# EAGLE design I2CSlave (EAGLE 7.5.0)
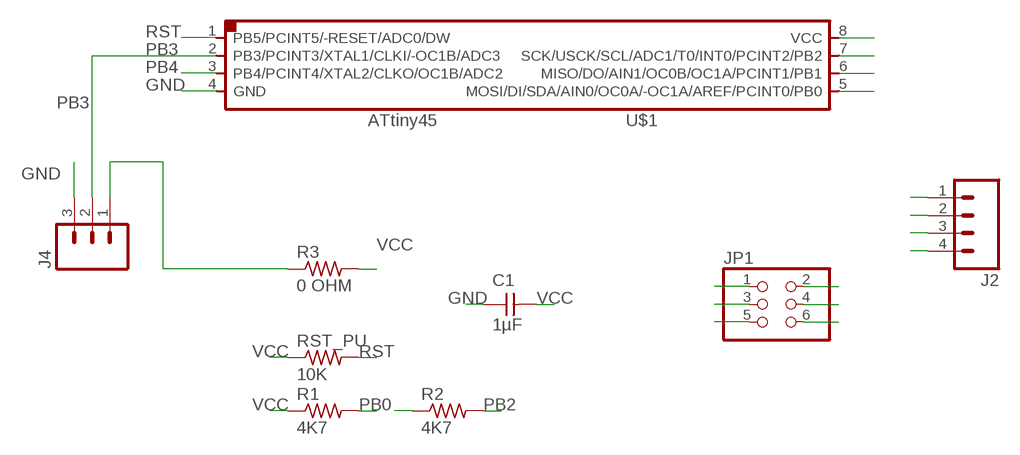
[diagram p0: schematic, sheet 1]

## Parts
C1  1µF  CAP-UNPOLARIZEDFAB  [C1206FAB]
J2  M04LONGPADS  [1X04_LONGPADS]
J4  M03LONGPADS  [1X03_LONGPADS]
JP1  PINHD-2X3-SMD  [2X03SMD]
R1  4K7  RES-US1206FAB  [R1206FAB]
R2  4K7  RES-US1206FAB  [R1206FAB]
R3  0 OHM  RES-US1206FAB  [R1206FAB]
RST_PU  10K  RES-US1206FAB  [R1206FAB]
U$1  ATTINY45SI  [SOIC8]

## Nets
GND: C1.1 J2.4 J4.3 JP1.6 U$1.4(GND)
MISO: JP1.1 U$1.6(MISO/DO/AIN1/OC0B/OC1A/PCINT1/PB1)
N$1: J4.1 R3.1
PB0: J2.2 JP1.4 R1.2 U$1.5(MOSI/DI/SDA/AIN0/OC0A/-OC1A/AREF/PCINT0/PB0)
PB2: J2.3 JP1.3 R2.2 U$1.7(SCK/USCK/SCL/ADC1/T0/INT0/PCINT2/PB2)
PB3: J4.2 U$1.2(PB3/PCINT3/XTAL1/CLKI/-OC1B/ADC3)
PB4: U$1.3(PB4/PCINT4/XTAL2/CLKO/OC1B/ADC2)
RST: JP1.5 RST_PU.2 U$1.1(PB5/PCINT5/-RESET/ADC0/DW)
VCC: C1.2 J2.1 JP1.2 R1.1 R2.1 R3.2 RST_PU.1 U$1.8(VCC)

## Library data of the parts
C1 = fab:CAP-UNPOLARIZED
J2 = SparkFun-Connectors:M04: Header 4 Standard 4-pin 0.1" header. Use with straight break away headers (SKU : PRT-00116), right angle break away headers (PRT-00553), swiss pins (PRT-00743), machine pins (PRT-00117), and female headers (PRT-00115). Molex polarized connector foot print use with SKU : PRT-08231 with associated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; PROD_ID: CONN-09696
J4 = SparkFun-Connectors:M03: Header 3 Standard 3-pin 0.1" header. Use with straight break away headers (SKU : PRT-00116), right angle break away headers (PRT-00553), swiss pins (PRT-00743), machine pins (PRT-00117), and female headers (PRT-00115). Molex polarized connector foot print use with SKU : PRT-08232 with associated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
JP1 = fab:PINHD-2X3-SMD: PIN HEADER
R1-R3 RST_PU = fab:RES-US: Resistor (US Symbol)
U$1 = fab:ATTINY45

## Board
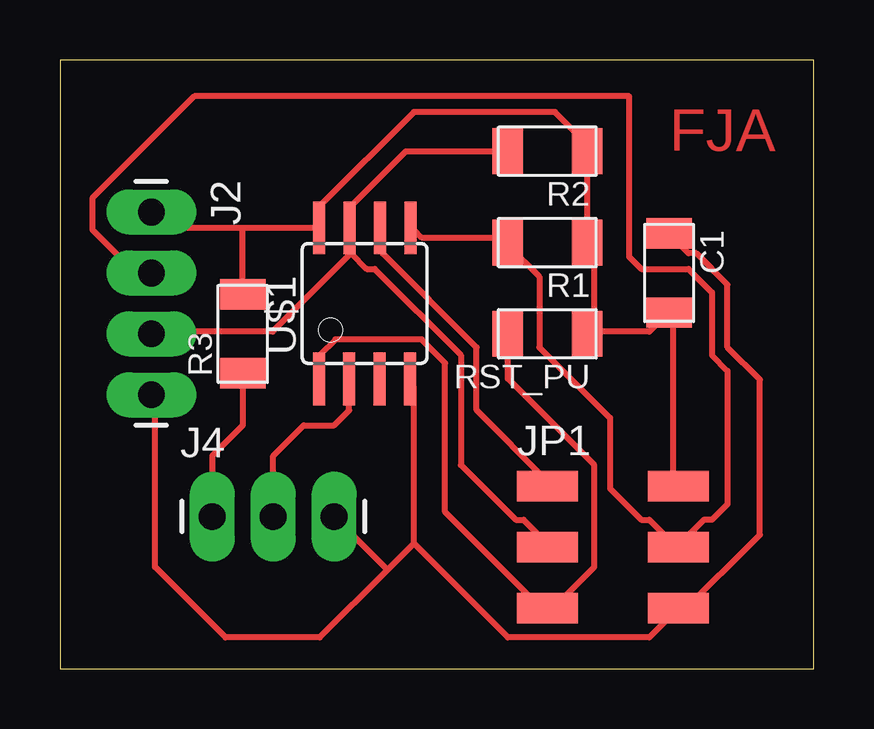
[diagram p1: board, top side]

Size 31.42 x 25.39 mm. Coordinates in mm from the lower left corner, seen from the top.
Outline: 0,0 31.42,0 31.42,25.39 0,25.39 0,0
Copper layers (1*16): Top 0.035mm / dielectric 1.5mm / Bottom 0.035mm
Design rules "default *": minimum track width 10mil, minimum drill 24mil, track to track 0.4mm, track to pad 0.4mm, pad to pad 0.4mm, via to via 0.4mm, smd to smd 8mil, copper to edge 40mil, drill to drill 8mil, minimum pad ring 10mil, minimum via ring 8mil, stop-mask expansion 4mil, vias tented up to drill 0mil, thermal gap 10mil

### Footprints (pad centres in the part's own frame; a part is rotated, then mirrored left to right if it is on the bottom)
C1206FAB = smd 1.27 x 1.905: 1 -1.651,0; 2 1.651,0
1X04_LONGPADS = drill 1.118 pad 1.88 long: 1 0,0; 2 2.54,0; 3 5.08,0; 4 7.62,0
1X03_LONGPADS = drill 1.118 pad 1.88 long: 1 0,0; 2 2.54,0; 3 5.08,0
2X03SMD = smd 2.54 x 1.27: 1 -2.54,2.54; 2 2.92,2.54; 3 -2.54,0; 4 2.92,0; 5 -2.54,-2.54; 6 2.92,-2.54
R1206FAB = smd 1.27 x 1.905: 1 -1.651,0; 2 1.651,0
SOIC8 = smd 0.5 x 2.2: 1 -1.905,-3.154; 2 -0.645,-3.154; 3 0.625,-3.154; 4 1.895,-3.154; 5 1.905,3.154; 6 0.635,3.154; 7 -0.635,3.154; 8 -1.905,3.154

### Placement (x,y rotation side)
C1  25.4,16.51 270 top
J2  3.81,19.05 270 top
J4  6.35,6.35 0 top
JP1  22.86,5.08 0 top
R1  20.32,17.78 180 top
R2  20.32,21.59 180 top
R3  7.62,13.97 90 top
RST_PU  20.32,13.97 180 top
U$1  12.7,15.24 0 top

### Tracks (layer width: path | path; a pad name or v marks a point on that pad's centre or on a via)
GND
  Top 0.254: C1.1 25.54,17.98 26.2,17.33 26.53,17.33 27.83,16.02 27.83,13.41 29.18,12.06 29.18,5.6 25.87,2.29 JP1.6 25.54,2.29 24.56,1.31 18.68,1.31 14.75,5.23 | 14.75,5.23 14.75,11.77 U$1.4 | 14.75,5.23 13.65,4.13 | 13.65,4.13 10.83,1.31 6.91,1.31 3.96,4.25 3.96,11.12 J2.4 | J4.3 13.65,4.13
MISO
  Top 0.254: U$1.6 13.45,18.31 13.45,17.33 17.37,13.41 17.37,10.79 20.31,7.85 JP1.1
N$1
  Top 0.254: R3.1 7.62,10.16 6.35,8.89 J4.1
PB0
  Top 0.254: U$1.5 14.75,18.31 15.08,17.98 18.35,17.98 R1.2 18.68,17.66 19.98,16.35 19.98,13.41 22.93,10.46 22.93,7.52 24.24,6.21 24.56,6.21 25.54,5.23 JP1.4 25.87,5.23 26.85,6.21 27.18,6.21 27.83,6.87 27.83,12.43 27.18,13.08 27.18,15.7 26.2,16.68 24.24,16.68 23.73,17.18 23.73,23.87 5.6,23.87 1.35,19.62 1.35,18.31 2.98,16.68 3.64,16.68 J2.2
PB2
  Top 0.254: R2.2 18.35,21.58 14.43,21.58 12.14,19.29 12.14,18.64 U$1.7 | 12.14,17.33 12.79,16.68 13.12,16.68 16.71,13.08 16.71,8.5 19,6.21 19.33,6.21 20.31,5.23 JP1.3 | 12.14,17.33 12.14,18.31 U$1.7 | 12.14,17.33 8.87,14.06 3.96,14.06 J2.3 | 12.14,17.33 U$1.7
PB3
  Top 0.254: J4.2 8.89,8.89 10.16,10.16 11.43,10.16 12.05,10.79 U$1.2
RST
  Top 0.254: RST_PU.2 18.68,13.73 18.68,12.1 22.27,8.5 22.27,4.25 20.64,2.62 JP1.5 20.31,2.29 16.06,6.54 16.06,12.75 15.08,13.73 11.48,13.73 10.83,13.08 10.83,12.1 U$1.1
VCC
  Top 0.254: J2.1 3.96,18.97 4.53,18.39 7.62,18.39 | 22.27,14.06 24.56,14.06 25.22,14.71 C1.2 25.54,14.71 25.54,7.85 JP1.2 | 22.27,14.06 22.27,17.66 R1.1 R2.1 21.95,21.91 20.64,23.22 14.75,23.22 10.83,19.29 10.83,18.64 U$1.8 7.62,18.39 | 22.27,14.06 RST_PU.1 | R3.2 7.62,18.39

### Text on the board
Top: FJA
